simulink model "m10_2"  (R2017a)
settings: Solver=ode45  StartTime=0.0  StopTime=30  MaxStep=0.1  RelTol=1e-3  AbsTol=1e-6
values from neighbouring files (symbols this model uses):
  beta = 5    [ini_mst.m]    (also in vdpini.m = sqrt(3))
  mi = 0.1    [vdpini.m]
  omega = 4    [ini_mst.m]    (also in vdpini.m = 1)
libraries: simulink x1

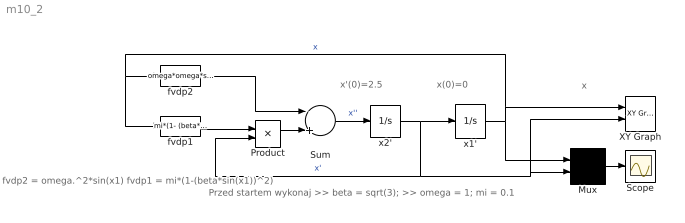
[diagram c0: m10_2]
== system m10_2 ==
  note: x
  note: Przed startem wykonaj >> beta = sqrt(3); >> omega = 1; mi = 0.1
  note: x(0)=0
  note: fvdp2 = omega.^2*sin(x1) fvdp1 = mi*(1-(beta*sin(x1))^2)
  note: x'(0)=2.5
  Mux : Mux  Inputs=2
  Product : Product
  Scope : Scope
  Sum : Sum  Inputs=-+
  XY Graph : simulink/Sinks/XY Graph  xmin=0  xmax=15.5  ymin=-2  ymax=3  st=-1
  fvdp1 : Fcn  Expr=mi*(1- (beta*sin(u[1]))*(beta*sin(u[1])))
  fvdp2 : Fcn  Expr=omega*omega*sin(u[1])
  x1' : Integrator
  x2' : Integrator  InitialCondition=2.5
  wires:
  fvdp2/1 -> Sum/1
  fvdp1/1 -> Product/1
  Product/1 -> Sum/2
  Sum/1 -> x2'/1  "x''"
  x2'/1 -> x1'/1, Product/2, XY Graph/2, Mux/2  "x'"
  x1'/1 -> fvdp2/1, fvdp1/1, XY Graph/1, Mux/1  "x"
  Mux/1 -> Scope/1
